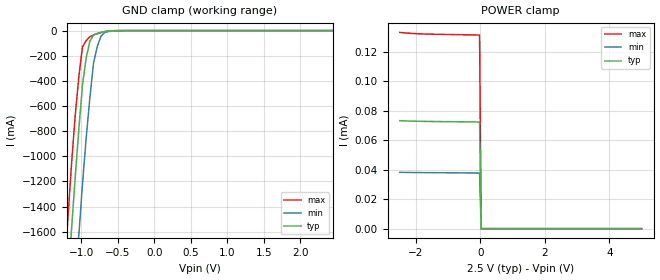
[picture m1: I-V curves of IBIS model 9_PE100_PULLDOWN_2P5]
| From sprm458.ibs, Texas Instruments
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|IDG09_PE100_NOPULLDOWN_2P75; BUFFER OPERATING IN NORMMAL MODE WITHOUT PULL
|DOWN
|   Model Cell 9_PE100_PULLDOWN_2P5
|IDG09_PE100_PULLDOWN_2P5
[Model]   9_PE100_PULLDOWN_2P5
Model_type   Input
Polarity   Non-Inverting
Vinl =  0.7V
Vinh =  1.7V
C_comp   1.348p   1.322p   1.399p
[Model Spec]
Vinl   0.7V   0.7V   0.7V
Vinh   1.7V   1.7V   1.7V
[Temperature Range]   25   125   -40
[Voltage Range]   2.5   2.3   2.7
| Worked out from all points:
|   GND clamp passes 1 mA (typ) near -0.54 V on its own axis
[POWER_clamp]
|   voltage   I(typ)   I(min)   I(max)
-2.5V     73.24uA    38.22uA    133.1uA
-1.742V   72.75uA    38.01uA    132uA
-25.25mV  72.31uA    37.72uA    131.3uA
25.25mV   0A         0A         0A
5V        0A         0A         0A
[GND_clamp]
|   voltage   I(typ)   I(min)   I(max)
-2.5V     -14.65A    -15.5A     -14.18A
-1.237V   -2.489A    -3.395A    -1.958A
-1.187V   -2.038A    -2.94A     -1.511A
-1.136V   -1.594A    -2.491A    -1.074A
-1.035V   -791.1mA   -1.633A    -371.5mA
-984.8mV  -434.4mA   -1.223A    -129.4mA
-934.3mV  -219.3mA   -857.5mA   -80.1mA
-883.8mV  -85.77mA   -536.6mA   -48.76mA
-833.3mV  -33.79mA   -260.3mA   -35.42mA
-782.8mV  -23.01mA   -128.3mA   -25.01mA
-681.8mV  -8.423mA   -15mA      -8.197mA
2.449V    72.28uA    37.75uA    131.2uA
